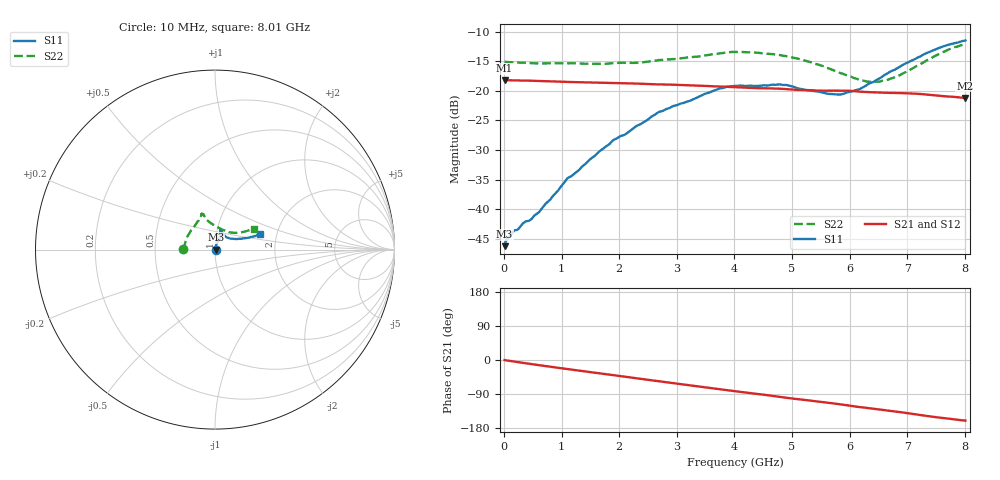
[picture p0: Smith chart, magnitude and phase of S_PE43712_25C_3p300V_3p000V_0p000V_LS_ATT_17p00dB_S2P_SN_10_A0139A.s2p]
! DEVICE ID: PE43712
! File Path: z:\PE43713\PE43713_CHAR_NOM_04292014\AMB\3p300\LS_ATT_17p00dB\PE43713_AMB_3p300V_3p000V_0p000V_LS_ATT_17p00dB_S2P_SN_10_A0139A.s2p
! Serial: 10
! Lot: A0139A
! Temp: 25C
! VDD: 3.300
! VSS: 0.000
! Control_Hi: 3.000
! Control_Lo: 0.000
! Attenuation Step: 17.00dB
! Port 1: RF1
! Port 2: RF2
! ThroughPath:1-2
! IDD: 0.0001464348
! ISS: -1.37e-007
#  Hz  S  RI  R  50
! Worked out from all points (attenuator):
!   801 points, 10 MHz to 8.01 GHz, reference 50 ohm
!   highest |S21| = -18.21 dB at 10 MHz (marker M1); lowest = -21.2 dB at 8 GHz (marker M2)
!   lowest |S11| = -46.3 dB at 10 MHz (marker M3), VSWR 1.01, Z = 50.5 + j0.0427 ohm
!   |S11| at or under -10 dB: start of sweep to end of sweep
!   |S22| runs from -18.6 to -12.2 dB; largest |S21 - S12| = 0.00044
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1e7  0.00485 0.000423  0.1229 -0.000582  0.123 -0.000568  -0.1759 0.00113
1.6e8  0.00596 0.00242  0.1223 -0.00799  0.1223 -0.008  -0.1736 0.0113
6e8  0.00556 0.00753  0.1176 -0.0281  0.1176 -0.0281  -0.1664 0.0358
1.09e9  0.00476 0.0173  0.1088 -0.0478  0.1089 -0.0478  -0.158 0.0634
1.35e9  0.00584 0.022  0.1033 -0.0571  0.1033 -0.0571  -0.1518 0.076
1.9e9  0.0117 0.0365  0.089 -0.0748  0.089 -0.0748  -0.1335 0.107
2.11e9  0.0142 0.0406  0.0828 -0.0808  0.0828 -0.0807  -0.1272 0.1162
2.68e9  0.0257 0.0607  0.0638 -0.0936  0.0638 -0.0936  -0.1016 0.1507
3.72e9  0.0323 0.0984  0.0252 -0.1057  0.0251 -0.1057  -0.0762 0.1916
4.01e9  0.0324 0.105  0.0144 -0.1064  0.0143 -0.1063  -0.0753 0.1995
4.79e9  0.0331 0.1083  -0.0132 -0.1031  -0.0132 -0.1032  -0.0621 0.1904
5.35e9  0.0442 0.0895  -0.0308 -0.0962  -0.0308 -0.0961  -0.0468 0.1664
5.64e9  0.0542 0.0769  -0.039 -0.0924  -0.039 -0.0924  -0.0286 0.1516
5.87e9  0.0639 0.0682  -0.0464 -0.0886  -0.0463 -0.0887  -0.0102 0.1395
6.17e9  0.0824 0.062  -0.0551 -0.0814  -0.0549 -0.0815  0.0188 0.122
6.38e9  0.1 0.061  -0.0595 -0.0767  -0.0593 -0.0767  0.0423 0.1106
6.68e9  0.1297 0.0595  -0.0662 -0.0696  -0.0661 -0.0696  0.0783 0.0975
6.99e9  0.1594 0.0629  -0.0729 -0.0612  -0.0728 -0.0611  0.1107 0.0932
7.37e9  0.1995 0.0704  -0.0787 -0.0487  -0.0786 -0.0486  0.1548 0.0986
7.72e9  0.232 0.0791  -0.0808 -0.038  -0.0807 -0.038  0.1947 0.1096
8e9  0.2502 0.0889  -0.0815 -0.03  -0.0814 -0.0301  0.2151 0.1165
8.01e9  0.2507 0.0896  -0.0816 -0.0298  -0.0814 -0.03  0.2158 0.1166
